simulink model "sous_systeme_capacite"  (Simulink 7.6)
settings: Solver=ode45  StartTime=0.0  StopTime=10.0  RelTol=1e-3
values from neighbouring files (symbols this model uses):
  R1 = 1e3    (= 1000)    [filtre_pbande.m]    (also in impedance_quartz.m = 30; Calcul_symbolique_RLC.m = 1)
  R2 = 10e3    (= 10000)    [filtre_pbande.m]    (also in Calcul_symbolique_RLC.m = 1; _startup.m = 100000)
libraries: elec_lib x2, fl_lib x2

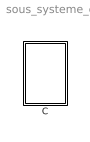
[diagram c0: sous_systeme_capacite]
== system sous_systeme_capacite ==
  C : Subsystem

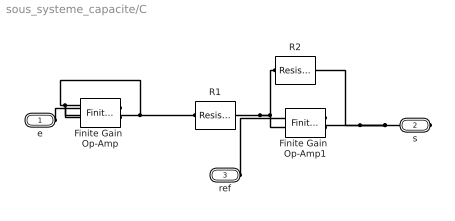
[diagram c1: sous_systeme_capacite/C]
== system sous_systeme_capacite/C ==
  Finite Gain  Op-Amp : elec_lib/Integrated Circuits/Finite Gain Op-Amp  DialogController=NetworkEngine.DynNeDlgSource  SystemSampleTime=-1  A=1000  Rin=1e+6 Ohm  Rout=100 Ohm  Vmin=-15 V  Vmax=15 V  LocalVarLogging=[]
  Finite Gain  Op-Amp1 : elec_lib/Integrated Circuits/Finite Gain Op-Amp  DialogController=NetworkEngine.DynNeDlgSource  SystemSampleTime=-1  A=1000  Rin=1e+6 Ohm  Rout=100 Ohm  Vmin=-15 V  Vmax=15 V  LocalVarLogging=[]
  R1 : fl_lib/Electrical/Electrical Elements/Resistor  DialogController=NetworkEngine.DynNeDlgSource  SystemSampleTime=-1  R=R1 Ohm  i_Log=off  v_Log=off  LocalVarNames=|i|v  LocalVarDescs=|i|v  LocalVarLogging=[0 0]
  R2 : fl_lib/Electrical/Electrical Elements/Resistor  DialogController=NetworkEngine.DynNeDlgSource  SystemSampleTime=-1  R=R2 Ohm  i_Log=off  v_Log=off  LocalVarNames=|i|v  LocalVarDescs=|i|v  LocalVarLogging=[0 0]
  e : PMIOPort  Port=1  Side=Left
  s : PMIOPort  Port=2  Side=Right
  ref : PMIOPort  Port=3  Side=Left
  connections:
  Finite Gain  Op-Amp/LConn2 -- Finite Gain  Op-Amp/RConn1 -- R1/LConn1
  Finite Gain  Op-Amp1/LConn2 -- R1/RConn1 -- R2/LConn1
  s/RConn1 -- Finite Gain  Op-Amp1/RConn1 -- R2/RConn1
  e/RConn1 -- Finite Gain  Op-Amp/LConn1
  ref/RConn1 -- Finite Gain  Op-Amp1/LConn1
